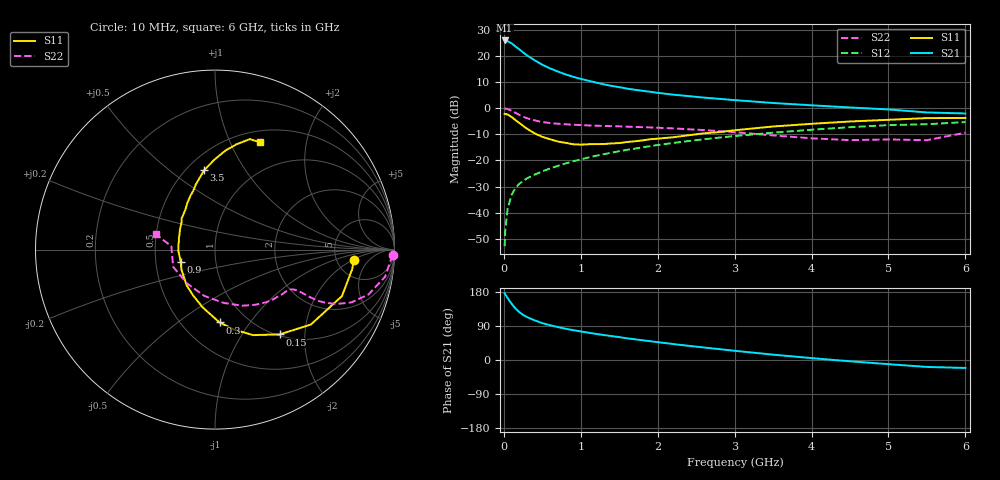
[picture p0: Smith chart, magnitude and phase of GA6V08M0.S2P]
! Infineon Technologies  Discrete & RF Semiconductors
! BF775
! Si NPN RF Bipolar Junction Transistor in SOT23
! VCE = 6 V  IC = 8 mA
! Common Emitter S-Parameters:  May  1996
# GHz  S  MA  R  50
!  f  S11  S21  S12  S22
! GHz  MAG  ANG  MAG  ANG  MAG  ANG  MAG  ANG
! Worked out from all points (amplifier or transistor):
!   36 points, 10 MHz to 6 GHz, reference 50 ohm
!   highest |S21| = 25.9 dB at 10 MHz (marker M1)
!   |S21| within 3 dB of that: start of sweep to 183.2 MHz
!   unconditionally stable (mu >= 1): 680.2 MHz to 3 GHz
!   at 250 MHz: K = 0.61, MSG = 24.6 dB, |S12| = -27.9 dB
!   at 1.4 GHz: K = 1.10, MAG = 10.8 dB, |S12| = -17.0 dB
!   at 6 GHz: K = 0.91, MSG = 1.6 dB, |S12| = -5.3 dB
!   S11 on the Smith chart (normalised r, x): 10 MHz: 7.35, -2.05; 150 MHz: 1.02, -1.49; 300 MHz: 0.75, -0.73; 900 MHz: 0.67, -0.10; 3.5 GHz: 0.61, +0.67; 6 GHz: 0.63, +1.30
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0.01  0.776 -4.1  19.66 176.2  0.0023 87.7  0.9898 -1.7
0.02  0.7724 -8.0  19.33 172.7  0.0049 83.6  0.9796 -3.7
0.05  0.7533 -20.1  18.95 163.2  0.012 80.4  0.9603 -9.0
0.1  0.678 -38.0  17.34 148.6  0.0219 72.2  0.891 -16.3
0.15  0.594 -52.7  15.15 136.1  0.0296 66.6  0.8144 -21.2
0.2  0.5215 -66.0  13.33 126.7  0.0358 64.0  0.7442 -24.0
0.25  0.4579 -76.6  11.63 119.0  0.0404 62.0  0.6846 -25.7
0.3  0.4069 -86.4  10.22 113.3  0.0454 61.2  0.6426 -26.4
0.4  0.329 -102.1  8.208 104.6  0.0536 61.4  0.5828 -26.6
0.5  0.2827 -115.7  6.751 97.3  0.0618 62.0  0.5425 -26.4
0.6  0.2544 -128.3  5.761 91.8  0.0703 62.6  0.5191 -26.4
0.7  0.2303 -139.1  5.02 87.0  0.0786 63.0  0.5042 -26.5
0.9  0.2041 -159.6  3.977 78.8  0.0962 63.4  0.4818 -27.4
1.1  0.2041 -177.7  3.331 72.1  0.1139 63.7  0.4674 -29.1
1.3  0.2059 168.4  2.847 65.9  0.1321 62.9  0.4564 -31.2
1.6  0.2252 150.3  2.366 57.3  0.1595 61.3  0.4423 -35.3
2.2  0.2774 126.5  1.811 42.2  0.2159 56.8  0.4102 -45.5
2.8  0.3486 110.4  1.506 28.7  0.2735 51.0  0.363 -58.7
3.5  0.4459 97.9  1.254 14.1  0.3395 42.9  0.3012 -80.6
4.5  0.5557 83.9  1.03 -3.4  0.4327 30.4  0.2445 -130.0
5.5  0.6455 72.5  0.827 -18.3  0.493 15.5  0.244 175.5
6  0.6481 67.2  0.791 -21.0  0.5412 11.3  0.3393 165.6
